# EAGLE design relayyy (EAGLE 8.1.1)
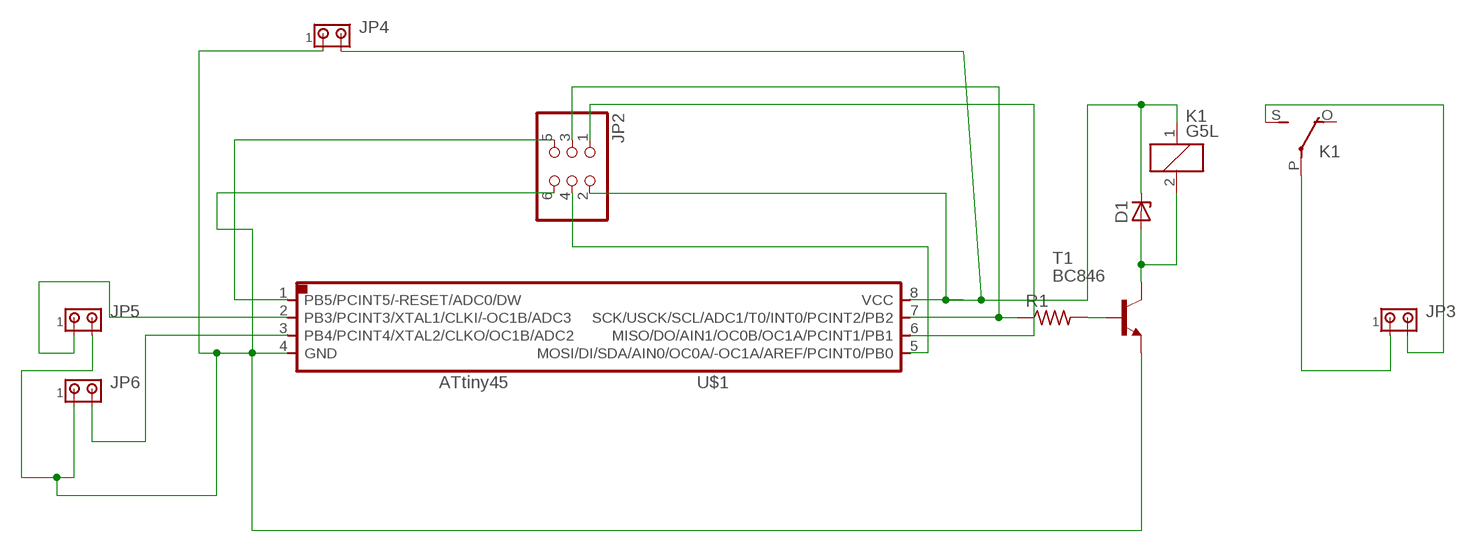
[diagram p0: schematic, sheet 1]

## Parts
D1  ZENER_DIODESOD123  [SOD123]
JP2  PINHD-2X3-SMD  [2X03SMD]
JP3  MTA02-156  [1X2MTA]
JP4  MTA02-156  [1X2MTA]
JP5  MTA02-156  [1X2MTA]
JP6  MTA02-156  [1X2MTA]
K1  G5L  [G5LE]
R1  RES-US1206  [R1206]
T1  BC846  [SOT23]
U$1  ATTINY45SI  [SOIC8]

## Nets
N$2: D1.CATHODE JP2.2 JP4.2 K1.1 U$1.8(VCC)
N$3: JP2.5 U$1.1(PB5/PCINT5/-RESET/ADC0/DW)
N$4: JP2.4 U$1.5(MOSI/DI/SDA/AIN0/OC0A/-OC1A/AREF/PCINT0/PB0)
N$5: JP2.3 R1.1 U$1.7(SCK/USCK/SCL/ADC1/T0/INT0/PCINT2/PB2)
N$6: JP2.1 U$1.6(MISO/DO/AIN1/OC0B/OC1A/PCINT1/PB1)
N$7: JP3.1 K1.P(2:P)
N$8: JP5.1 U$1.2(PB3/PCINT3/XTAL1/CLKI/-OC1B/ADC3)
N$9: D1.ANODE K1.2 T1.3(C)
N$10: R1.2 T1.1(B)
N$11: JP3.2 K1.S(2:S)
N$12: JP6.2 U$1.3(PB4/PCINT4/XTAL2/CLKO/OC1B/ADC2)
N$13: JP2.6 JP4.1 JP5.2 JP6.1 T1.2(E) U$1.4(GND)
Unconnected: K1.O(2:O)

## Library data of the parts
D1 = fab:ZENER_DIODE: zener diode
JP2 = fab:PINHD-2X3-SMD: PIN HEADER
JP3-JP6 = con-amp:MTA02-156: AMP connector
K1 = relay:G5L: RELAY 1 x switch, 10 A/120 V AC, 8 A/30 V ADC, Omron; OC_FARNELL: unknown; OC_NEWARK: unknown
R1 = fab:RES-US: Resistor (US Symbol)
T1 = transistor:BC846: NPN TRANSISTOR
U$1 = fab:ATTINY45

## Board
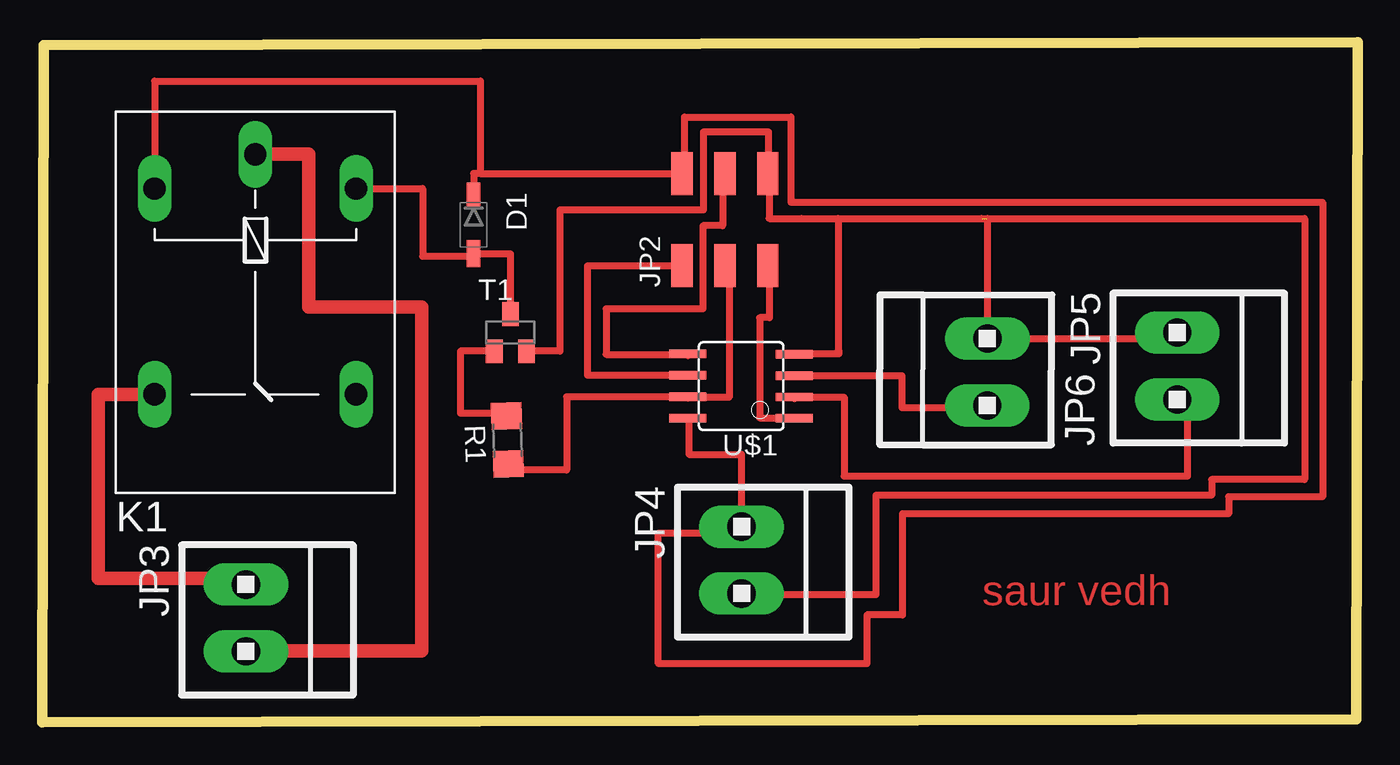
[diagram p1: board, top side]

Size 77.93 x 40.33 mm. Coordinates in mm from the lower left corner, seen from the top.
Outline: 0,0 77.83,0.18 77.93,40.32 0.1,40.15 0,0
Copper layers (1*16): Top 0.035mm / dielectric 1.5mm / Bottom 0.035mm
Design rules "default": minimum track width 10mil, minimum drill 24mil, track to track 8mil, track to pad 8mil, pad to pad 8mil, via to via 8mil, smd to smd 8mil, copper to edge 40mil, drill to drill 8mil, minimum pad ring 10mil, minimum via ring 8mil, stop-mask expansion 4mil, vias tented up to drill 0mil, thermal gap 10mil

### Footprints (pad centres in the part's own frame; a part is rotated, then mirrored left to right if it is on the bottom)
SOD123 = smd 1.6 x 0.8: ANODE 1.7,0; CATHODE -1.7,0
2X03SMD = smd 2.54 x 1.27: 1 -2.54,2.54; 2 2.92,2.54; 3 -2.54,0; 4 2.92,0; 5 -2.54,-2.54; 6 2.92,-2.54
1X2MTA = drill 1.676 long: 1 1.981,0; 2 -1.981,0
G5LE = drill 1.321 long: 1 -7.493,-5.969; 2 -7.493,5.969; O 4.699,5.969; P -9.525,0; S 4.699,-5.969
R1206 = smd 1.6 x 1.803: 1 -1.422,0; 2 1.422,0
SOT23 = smd 1 x 1.4: 1 -0.95,-1.1; 2 0.95,-1.1; 3 0,1.1
SOIC8 = smd 0.5 x 2.2: 1 -1.905,-3.154; 2 -0.645,-3.154; 3 0.625,-3.154; 4 1.895,-3.154; 5 1.905,3.154; 6 0.635,3.154; 7 -0.635,3.154; 8 -1.905,3.154

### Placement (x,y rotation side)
D1  25.55,29.49 270 top
JP2  40.44,29.62 90 top
JP3  12.06,6.2 270 top
JP4  41.43,9.63 270 top
JP5  67.23,21.13 270 top
JP6  55.98,20.78 89.9 top
K1  12.62,24.16 270 top
R1  27.56,16.74 92 top
T1  27.74,23.11 0 top
U$1  41.4,19.94 90 top

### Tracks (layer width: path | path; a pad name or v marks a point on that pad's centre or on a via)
N$2
  Top 0.406: 37.95,18.03 U$1.8 38.3,18.03 38.3,15.9 41.43,15.9 JP4.2 41.43,11.79 42.29,11.79 42.29,11.23 36.5,11.23 36.5,3.48 48.84,3.48 48.84,6.38 50.95,6.38 50.95,12.37 70.28,12.37 70.28,13.39 75.84,13.39 75.84,30.84 44.35,30.84 44.35,35.89 38.05,35.89 38.05,32.54 JP2.2 | 37.9,33.22 JP2.2 | JP2.2 38.15,32.54 | 25.55,31.06 D1.CATHODE 25.55,32.54 25.96,32.54 | 25.96,32.54 JP2.2 | K1.1 6.66,38.02 25.96,38.02 25.96,32.54
N$3
  Top 0.406: U$1.1 44.56,18.06 42.49,18.06 42.49,24 43.08,24 43.08,27.08 JP2.5
N$4
  Top 0.406: 38.25,21.74 U$1.5 38.25,21.82 33.4,21.82 33.4,24.51 39.14,24.51 39.14,29.44 40.31,29.44 40.31,32.54 JP2.4 | 40.49,32.54 JP2.4 | JP2.4 40.46,32.54
N$5
  Top 0.406: JP2.3 40.69,27.08 40.69,19.28 38.25,19.28 U$1.7 | 38.25,19.23 U$1.7 | U$1.7 31.06,19.3 31.06,14.96 27.61,14.96 R1.1
N$6
  Top 0.406: JP2.1 32.31,27.08 32.31,20.57 U$1.6
N$7
  Top 0.406: 12.57,4.24 12.57,3.96 12.06,3.96 JP3.1
  Top 0.813: K1.P 15.8,33.68 15.8,24.61 22.48,24.61 22.48,4.24 12.57,4.24
N$8
  Top 0.406: 67.84,19.15 JP5.1 | 67.84,19.15 68.35,19.15 | 44.56,19.2 U$1.2 47.5,19.29 47.5,14.6 67.84,14.6 67.84,19.15
N$9
  Top 0.406: T1.3 27.74,27.79 D1.ANODE 25.55,27.63 22.53,27.63 22.53,31.65 K1.2
N$10
  Top 0.406: T1.1 24.77,22.01 24.77,18.34 27.51,18.34 R1.2
N$11
  Top 0.406: 12.32,8.53 12.32,7.59 12.06,7.59 JP3.2
  Top 0.813: K1.S 3.33,19.46 3.33,8.53 12.32,8.53
N$12
  Top 0.406: U$1.3 50.93,20.56 50.93,18.67 55.93,18.67 JP6.2
N$13  (1 unrouted)
  Top 0.406: JP6.1 67.23,22.76 JP5.2 | JP6.1 55.96,22.76 | 44.75,21.83 U$1.4 47.19,21.84 47.19,22.02 47.14,22.02 47.14,29.87 44.98,29.87 | 42.98,32.33 JP2.6 | JP2.6 42.75,32.54 | T1.2 30.66,22.01 30.66,30.38 39.17,30.38 39.17,35 43.03,35 43.03,32.54 JP2.6 | JP2.6 43.05,32.54 43.05,29.87 44.98,29.87 | 44.98,29.87 55.98,29.87 JP6.1 | 55.65,29.87 74.78,29.87 74.78,14.4 69.27,14.4 69.27,13.46 49.38,13.46 49.38,7.57 40.84,7.57 40.84,7.72 41.43,7.72 JP4.1

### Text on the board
Top: saur vedh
